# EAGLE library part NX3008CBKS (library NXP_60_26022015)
30 / 30 V, 350 / 200 mA N/P-channel Trench MOSFET Complementary N/P-channel enhancement mode Field-Effect Transistor (FET) in very small SOT363 (SC-88) Surface-Mounted Device (SMD) plastic package using Trench MOSFET technology AAL Eindhoven MK
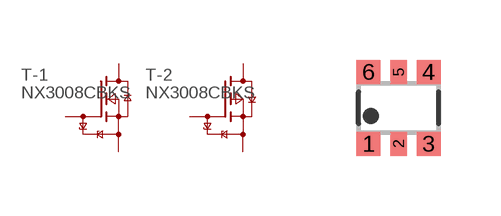
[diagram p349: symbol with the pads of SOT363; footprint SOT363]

Designator prefix T; gates -2=P-MOSFER-TR -1=N-MOSFET-ESD

## NX3008CBKS  [SOT363]
1  -1:S  pas
2  -1:G  pas
3  -2:D  pas
4  -2:S  pas
5  -2:G  pas
6  -1:D  pas

## Footprint SOT363 (pad centres in mm)
SOT363 Plastic surface-mounted package; 6 leads JEDEC: -- IEC: -- JEITA: SC-88
smd 0.6 x 0.6: 1 -0.75,-0.9; 3 0.75,-0.9; 4 0.75,0.9; 6 -0.75,0.9
smd 0.4 x 0.6: 2 0,-0.9; 5 0,0.9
